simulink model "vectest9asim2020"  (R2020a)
settings: Solver=FixedStepAuto  StartTime=0.0  StopTime=t(end)  FixedStep=dt  RelTol=1e-3  EnableMultiTasking=on
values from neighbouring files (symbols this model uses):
  arm = vectest9kinematics(arm,ind)    [vectest10demo2021.m]    (also in vectest11ademo2021.m; vectest11demo2021.m; vectest9ademo2.m = vectest9kinematics3(arm,ind); vectest9asim2020demo.m = vectest9kinematics3(arm,ind))
  dt = 0.001    [vectest9ademo2.m]    (also in vectest9asim2020demo.m; mobile10demo.m = 0.1; mobile2demo2021.m = 1)
undefined symbols (not defined in the file or in its folder): deg, kg, m, N, s, X, Y, Z
libraries: sm_lib x18, nesl_utility x12

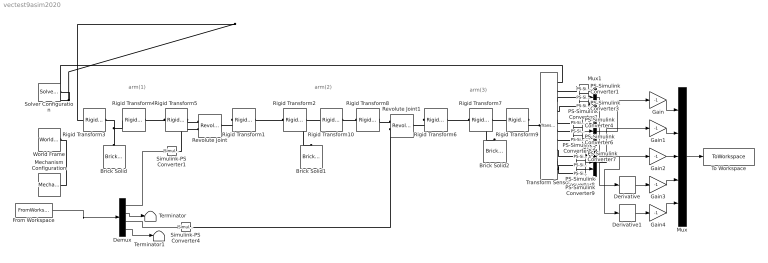
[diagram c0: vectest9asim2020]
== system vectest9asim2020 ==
  note: arm(1)
  note: arm(2)
  note: arm(3)
  Brick Solid : sm_lib/Body Elements/Brick Solid  GraphicAmbientColor=[0.15 0.15 0.15 1.0]  BasedOnType=Density  BrickDimensions=arm(1).l+[0.1;0.1;0]  BrickDimensionUnits=m  CenterOfMass=[0 0 0]  CenterOfMassUnits=m  GraphicDiffuseColor=[0.5 0.5 0.5]  Density=0  DensityUnits=kg/m^3  DoExposeReferenceFrame=on  GraphicEmissiveColor=[0.0 0.0 0.0 1.0]  ExportEntireGeometry=off  SerializedFrames=<Frames/>  MarkerShape=Sphere  MarkerSize=10  GraphicType=FromGeometry  InertiaType=CalculateFromGeometry  Mass=1  MassUnits=kg  MomentsOfInertia=[1 1 1]  MomentsOfInertiaUnits=kg*m^2  GraphicOpacity=1.0  ProductsOfInertia=[0 0 0]  ProductsOfInertiaUnits=kg*m^2  GraphicShininess=75  GraphicSpecularColor=[0.5 0.5 0.5 1.0]  GraphicVisPropType=SimpleVisualProperties
  Brick Solid1 : sm_lib/Body Elements/Brick Solid  GraphicAmbientColor=[0.15 0.15 0.15 1.0]  BasedOnType=Density  BrickDimensions=arm(2).l+[0.1;0.1;0]  BrickDimensionUnits=m  CenterOfMass=[0 0 0]  CenterOfMassUnits=m  GraphicDiffuseColor=[0.5 0.5 0.5]  Density=0  DensityUnits=kg/m^3  DoExposeReferenceFrame=on  GraphicEmissiveColor=[0.0 0.0 0.0 1.0]  ExportEntireGeometry=off  SerializedFrames=<Frames/>  MarkerShape=Sphere  MarkerSize=10  GraphicType=FromGeometry  InertiaType=CalculateFromGeometry  Mass=1  MassUnits=kg  MomentsOfInertia=[1 1 1]  MomentsOfInertiaUnits=kg*m^2  GraphicOpacity=1.0  ProductsOfInertia=[0 0 0]  ProductsOfInertiaUnits=kg*m^2  GraphicShininess=75  GraphicSpecularColor=[0.5 0.5 0.5 1.0]  GraphicVisPropType=SimpleVisualProperties
  Brick Solid2 : sm_lib/Body Elements/Brick Solid  GraphicAmbientColor=[0.15 0.15 0.15 1.0]  BasedOnType=Density  BrickDimensions=arm(3).l+[0.1;0.1;0]  BrickDimensionUnits=m  CenterOfMass=[0 0 0]  CenterOfMassUnits=m  GraphicDiffuseColor=[0.5 0.5 0.5]  Density=0  DensityUnits=kg/m^3  DoExposeReferenceFrame=on  GraphicEmissiveColor=[0.0 0.0 0.0 1.0]  ExportEntireGeometry=off  SerializedFrames=<Frames/>  MarkerShape=Sphere  MarkerSize=10  GraphicType=FromGeometry  InertiaType=PointMass  Mass=0  MassUnits=kg  MomentsOfInertia=[1 1 1]  MomentsOfInertiaUnits=kg*m^2  GraphicOpacity=1.0  ProductsOfInertia=[0 0 0]  ProductsOfInertiaUnits=kg*m^2  GraphicShininess=75  GraphicSpecularColor=[0.5 0.5 0.5 1.0]  GraphicVisPropType=SimpleVisualProperties
  Demux : Demux  Outputs=[1,2,1,2]
  Derivative : Derivative
  Derivative1 : Derivative
  From Workspace : FromWorkspace  VariableName=simin  SampleTime=dt
  Gain{,1..4} (5 alike) : Gain  Gain=-1
  Mechanism Configuration : sm_lib/Utilities/Mechanism Configuration  UniformGravity=Constant  GravityVector=[0 0 0]  GravityUnits=m/s^2  LinearizationDelta=0.001
  Mux : Mux  Inputs=[3,3,3,3,3]
  Mux1 : Mux  Inputs=[1,1,1]
  Mux2 : Mux  Inputs=[1,1,1]
  Mux3 : Mux  Inputs=[1,1,1]
  PS-Simulink Converter{1..9} (9 alike) : nesl_utility/PS-Simulink Converter  PhysicalDomain=network_engine_domain  SubClassName=ps_output  LeftPortType=input  RightPortType=output  PseudoPeriodic=off  Frequencies=[]  Unit=inherit  AffineConversion=off
  Revolute Joint : sm_lib/Joints/Revolute Joint  JointMode=Normal  SenseConstraintForce=off  SenseConstraintForceX=off  SenseConstraintForceY=off  SenseConstraintForceZ=off  SenseConstraintTorque=off  SenseConstraintTorqueX=off  SenseConstraintTorqueY=off  SenseConstraintTorqueZ=off  SenseTotalForce=off  SenseTotalForceX=off  SenseTotalForceY=off  SenseTotalForceZ=off  SenseTotalTorque=off  SenseTotalTorqueX=off  SenseTotalTorqueY=off  SenseTotalTorqueZ=off  CompositeWrenchDir=FollowerOnBase  CompositeWrenchFrame=BaseFrame  EquilibriumPosition=0  EquilibriumPositionUnits=rad  SpringStiffness=0  SpringStiffnessUnits=N*m/deg  DampingCoefficient=0  DampingCoefficientUnits=N*m/(deg/s)  TorqueActuationMode=ComputedTorque  MotionActuationMode=InputMotion  SensePosition=off  SenseVelocity=off  SenseAcceleration=off  SenseTorqueForce=off  SenseLowerLimitTorqueForce=off  SenseUpperLimitTorqueForce=off  LowerLimitSpecify=off  LowerLimitBound=-90  LowerLimitBoundUnits=deg  LowerLimitStiffness=1e4  LowerLimitStiffnessUnits=N*m/deg  LowerLimitDamping=10  LowerLimitDampingUnits=N*m/(deg/s)  LowerLimitTransitionRegionWidth=0.1  LowerLimitTransitionRegionWidthUnits=deg  UpperLimitSpecify=off  UpperLimitBound=90  UpperLimitBoundUnits=deg  UpperLimitStiffness=1e4  UpperLimitStiffnessUnits=N*m/deg  UpperLimitDamping=10  UpperLimitDampingUnits=N*m/(deg/s)  UpperLimitTransitionRegionWidth=0.1  UpperLimitTransitionRegionWidthUnits=deg  PositionTargetSpecify=off  PositionTargetPriority=High  PositionTargetValue=0  PositionTargetValueUnits=deg  VelocityTargetSpecify=off  VelocityTargetPriority=High  VelocityTargetValue=0  VelocityTargetValueUnits=deg/s
  Revolute Joint1 : sm_lib/Joints/Revolute Joint  JointMode=Normal  SenseConstraintForce=off  SenseConstraintForceX=off  SenseConstraintForceY=off  SenseConstraintForceZ=off  SenseConstraintTorque=off  SenseConstraintTorqueX=off  SenseConstraintTorqueY=off  SenseConstraintTorqueZ=off  SenseTotalForce=off  SenseTotalForceX=off  SenseTotalForceY=off  SenseTotalForceZ=off  SenseTotalTorque=off  SenseTotalTorqueX=off  SenseTotalTorqueY=off  SenseTotalTorqueZ=off  CompositeWrenchDir=FollowerOnBase  CompositeWrenchFrame=BaseFrame  EquilibriumPosition=0  EquilibriumPositionUnits=rad  SpringStiffness=0  SpringStiffnessUnits=N*m/deg  DampingCoefficient=0  DampingCoefficientUnits=N*m/(deg/s)  TorqueActuationMode=ComputedTorque  MotionActuationMode=InputMotion  SensePosition=off  SenseVelocity=off  SenseAcceleration=off  SenseTorqueForce=off  SenseLowerLimitTorqueForce=off  SenseUpperLimitTorqueForce=off  LowerLimitSpecify=off  LowerLimitBound=-90  LowerLimitBoundUnits=deg  LowerLimitStiffness=1e4  LowerLimitStiffnessUnits=N*m/deg  LowerLimitDamping=10  LowerLimitDampingUnits=N*m/(deg/s)  LowerLimitTransitionRegionWidth=0.1  LowerLimitTransitionRegionWidthUnits=deg  UpperLimitSpecify=off  UpperLimitBound=90  UpperLimitBoundUnits=deg  UpperLimitStiffness=1e4  UpperLimitStiffnessUnits=N*m/deg  UpperLimitDamping=10  UpperLimitDampingUnits=N*m/(deg/s)  UpperLimitTransitionRegionWidth=0.1  UpperLimitTransitionRegionWidthUnits=deg  PositionTargetSpecify=off  PositionTargetPriority=High  PositionTargetValue=0  PositionTargetValueUnits=deg  VelocityTargetSpecify=off  VelocityTargetPriority=High  VelocityTargetValue=0  VelocityTargetValueUnits=deg/s
  Rigid Transform1 : sm_lib/Frames and Transforms/Rigid Transform  TranslationMethod=None  TranslationStandardOffset=0  TranslationLengthUnit=m  TranslationStandardAxis=+Z  TranslationCartesianOffset=[0 0 0]  TranslationROffset=0  TranslationROffsetUnits=m  TranslationZOffset=0  TranslationZOffsetUnits=m  TranslationThetaOffset=0  TranslationThetaOffsetUnits=deg  RotationMethod=StandardAxis  RotationAngleUnits=deg  RotationStandardAxis=+Y  RotationAngle=-90  RotationArbitraryAxis=[0 0 1]  FollAlignAxisA=+X  BaseAlignAxisA=+Y  FollAlignAxisB=+Y  BaseAlignAxisB=+Z  RotationSequenceAxes=FollowerAxes  RotationSequence=XYX  RotationSequenceAngles=[0 0 0]  RotationSequenceAnglesUnits=deg  RotationMatrix=[1 0 0; 0 1 0; 0 0 1]
  Rigid Transform10 : sm_lib/Frames and Transforms/Rigid Transform  TranslationMethod=Cartesian  TranslationStandardOffset=1  TranslationLengthUnit=m  TranslationStandardAxis=+Z  TranslationCartesianOffset=arm(2).l/2  TranslationROffset=0  TranslationROffsetUnits=m  TranslationZOffset=0  TranslationZOffsetUnits=m  TranslationThetaOffset=0  TranslationThetaOffsetUnits=deg  RotationMethod=None  RotationAngleUnits=deg  RotationStandardAxis=+Y  RotationAngle=-90  RotationArbitraryAxis=[0 0 1]  FollAlignAxisA=+X  BaseAlignAxisA=+Y  FollAlignAxisB=+Y  BaseAlignAxisB=+Z  RotationSequenceAxes=FollowerAxes  RotationSequence=XYX  RotationSequenceAngles=[0 0 0]  RotationSequenceAnglesUnits=deg  RotationMatrix=[1 0 0; 0 1 0; 0 0 1]
  Rigid Transform2 : sm_lib/Frames and Transforms/Rigid Transform  TranslationMethod=Cartesian  TranslationStandardOffset=1  TranslationLengthUnit=m  TranslationStandardAxis=+Z  TranslationCartesianOffset=arm(2).l/2  TranslationROffset=0  TranslationROffsetUnits=m  TranslationZOffset=0  TranslationZOffsetUnits=m  TranslationThetaOffset=0  TranslationThetaOffsetUnits=deg  RotationMethod=None  RotationAngleUnits=deg  RotationStandardAxis=+Y  RotationAngle=-90  RotationArbitraryAxis=[0 0 1]  FollAlignAxisA=+X  BaseAlignAxisA=+Y  FollAlignAxisB=+Y  BaseAlignAxisB=+Z  RotationSequenceAxes=FollowerAxes  RotationSequence=XYX  RotationSequenceAngles=[0 0 0]  RotationSequenceAnglesUnits=deg  RotationMatrix=[1 0 0; 0 1 0; 0 0 1]
  Rigid Transform3 : sm_lib/Frames and Transforms/Rigid Transform  TranslationMethod=Cartesian  TranslationStandardOffset=0  TranslationLengthUnit=m  TranslationStandardAxis=+Z  TranslationCartesianOffset=arm(1).l/2  TranslationROffset=0  TranslationROffsetUnits=m  TranslationZOffset=0  TranslationZOffsetUnits=m  TranslationThetaOffset=0  TranslationThetaOffsetUnits=deg  RotationMethod=None  RotationAngleUnits=deg  RotationStandardAxis=+Y  RotationAngle=-90  RotationArbitraryAxis=[0 0 1]  FollAlignAxisA=+X  BaseAlignAxisA=+Y  FollAlignAxisB=+Y  BaseAlignAxisB=+Z  RotationSequenceAxes=FollowerAxes  RotationSequence=XYX  RotationSequenceAngles=[0 0 0]  RotationSequenceAnglesUnits=deg  RotationMatrix=[1 0 0; 0 1 0; 0 0 1]
  Rigid Transform4 : sm_lib/Frames and Transforms/Rigid Transform  TranslationMethod=Cartesian  TranslationStandardOffset=0  TranslationLengthUnit=m  TranslationStandardAxis=+Z  TranslationCartesianOffset=arm(1).l/2  TranslationROffset=0  TranslationROffsetUnits=m  TranslationZOffset=0  TranslationZOffsetUnits=m  TranslationThetaOffset=0  TranslationThetaOffsetUnits=deg  RotationMethod=None  RotationAngleUnits=deg  RotationStandardAxis=+Y  RotationAngle=-90  RotationArbitraryAxis=[0 0 1]  FollAlignAxisA=+X  BaseAlignAxisA=+Y  FollAlignAxisB=+Y  BaseAlignAxisB=+Z  RotationSequenceAxes=FollowerAxes  RotationSequence=XYX  RotationSequenceAngles=[0 0 0]  RotationSequenceAnglesUnits=deg  RotationMatrix=[1 0 0; 0 1 0; 0 0 1]
  Rigid Transform5 : sm_lib/Frames and Transforms/Rigid Transform  TranslationMethod=None  TranslationStandardOffset=0  TranslationLengthUnit=m  TranslationStandardAxis=+Z  TranslationCartesianOffset=[0 0 0.5]  TranslationROffset=0  TranslationROffsetUnits=m  TranslationZOffset=0  TranslationZOffsetUnits=m  TranslationThetaOffset=0  TranslationThetaOffsetUnits=deg  RotationMethod=StandardAxis  RotationAngleUnits=deg  RotationStandardAxis=+Y  RotationAngle=90  RotationArbitraryAxis=[0 0 1]  FollAlignAxisA=+X  BaseAlignAxisA=+Y  FollAlignAxisB=+Y  BaseAlignAxisB=+Z  RotationSequenceAxes=FollowerAxes  RotationSequence=XYX  RotationSequenceAngles=[0 0 0]  RotationSequenceAnglesUnits=deg  RotationMatrix=[1 0 0; 0 1 0; 0 0 1]
  Rigid Transform6 : sm_lib/Frames and Transforms/Rigid Transform  TranslationMethod=None  TranslationStandardOffset=0  TranslationLengthUnit=m  TranslationStandardAxis=+Z  TranslationCartesianOffset=[0 0 0]  TranslationROffset=0  TranslationROffsetUnits=m  TranslationZOffset=0  TranslationZOffsetUnits=m  TranslationThetaOffset=0  TranslationThetaOffsetUnits=deg  RotationMethod=StandardAxis  RotationAngleUnits=deg  RotationStandardAxis=-X  RotationAngle=-90  RotationArbitraryAxis=[0 0 1]  FollAlignAxisA=+X  BaseAlignAxisA=+Y  FollAlignAxisB=+Y  BaseAlignAxisB=+Z  RotationSequenceAxes=FollowerAxes  RotationSequence=XYX  RotationSequenceAngles=[0 0 0]  RotationSequenceAnglesUnits=deg  RotationMatrix=[1 0 0; 0 1 0; 0 0 1]
  Rigid Transform7 : sm_lib/Frames and Transforms/Rigid Transform  TranslationMethod=Cartesian  TranslationStandardOffset=1  TranslationLengthUnit=m  TranslationStandardAxis=+Z  TranslationCartesianOffset=arm(3).l/2  TranslationROffset=0  TranslationROffsetUnits=m  TranslationZOffset=0  TranslationZOffsetUnits=m  TranslationThetaOffset=0  TranslationThetaOffsetUnits=deg  RotationMethod=None  RotationAngleUnits=deg  RotationStandardAxis=+Y  RotationAngle=-90  RotationArbitraryAxis=[0 0 1]  FollAlignAxisA=+X  BaseAlignAxisA=+Y  FollAlignAxisB=+Y  BaseAlignAxisB=+Z  RotationSequenceAxes=FollowerAxes  RotationSequence=XYX  RotationSequenceAngles=[0 0 0]  RotationSequenceAnglesUnits=deg  RotationMatrix=[1 0 0; 0 1 0; 0 0 1]
  Rigid Transform8 : sm_lib/Frames and Transforms/Rigid Transform  TranslationMethod=None  TranslationStandardOffset=0  TranslationLengthUnit=m  TranslationStandardAxis=+Z  TranslationCartesianOffset=[0 0 0.5]  TranslationROffset=0  TranslationROffsetUnits=m  TranslationZOffset=0  TranslationZOffsetUnits=m  TranslationThetaOffset=0  TranslationThetaOffsetUnits=deg  RotationMethod=StandardAxis  RotationAngleUnits=deg  RotationStandardAxis=-X  RotationAngle=90  RotationArbitraryAxis=[0 0 1]  FollAlignAxisA=+X  BaseAlignAxisA=+Y  FollAlignAxisB=+Y  BaseAlignAxisB=+Z  RotationSequenceAxes=FollowerAxes  RotationSequence=XYX  RotationSequenceAngles=[0 0 0]  RotationSequenceAnglesUnits=deg  RotationMatrix=[1 0 0; 0 1 0; 0 0 1]
  Rigid Transform9 : sm_lib/Frames and Transforms/Rigid Transform  TranslationMethod=Cartesian  TranslationStandardOffset=1  TranslationLengthUnit=m  TranslationStandardAxis=+Z  TranslationCartesianOffset=arm(3).l/2  TranslationROffset=0  TranslationROffsetUnits=m  TranslationZOffset=0  TranslationZOffsetUnits=m  TranslationThetaOffset=0  TranslationThetaOffsetUnits=deg  RotationMethod=None  RotationAngleUnits=deg  RotationStandardAxis=+Y  RotationAngle=-90  RotationArbitraryAxis=[0 0 1]  FollAlignAxisA=+X  BaseAlignAxisA=+Y  FollAlignAxisB=+Y  BaseAlignAxisB=+Z  RotationSequenceAxes=FollowerAxes  RotationSequence=XYX  RotationSequenceAngles=[0 0 0]  RotationSequenceAnglesUnits=deg  RotationMatrix=[1 0 0; 0 1 0; 0 0 1]
  Simulink-PS Converter1 : nesl_utility/Simulink-PS Converter  PhysicalDomain=network_engine_domain  SubClassName=ps_input  LeftPortType=input  RightPortType=output  PseudoPeriodic=off  Frequencies=[]  NoiseDistribution=none  NoiseParameters=[]  Unit=1  AffineConversion=off  FilteringAndDerivatives=filter  SimscapeFilterOrder=2  InputFilterTimeConstant=0.001  UdotUserProvided=0
  Simulink-PS Converter4 : nesl_utility/Simulink-PS Converter  PhysicalDomain=network_engine_domain  SubClassName=ps_input  LeftPortType=input  RightPortType=output  PseudoPeriodic=off  Frequencies=[]  NoiseDistribution=none  NoiseParameters=[]  Unit=1  AffineConversion=off  FilteringAndDerivatives=filter  SimscapeFilterOrder=2  InputFilterTimeConstant=0.001  UdotUserProvided=0
  Solver Configuration : nesl_utility/Solver Configuration  PhysicalDomain=network_engine_domain  SubClassName=solver  LeftPortType=input  RightPortType=generic  Tones=[]  Harmonics=[]  SimulateNoise=off  Profile=off  UseLocalSampling=off  EnableSwitchedLinearOptims=on  FrequencyDomain=off  UseCCode=off  RelTol=0.001  AbsTol=1e-06  MinStep=1e-09  ToWorkspace=off  RevertToSquareIcSolve=off  NumHomotopyIterations=100  PhasorMode=off  PhasorModeNumHarmonics=1  DoDC=off  ResidualTolerance=1e-09  UseLocalSolver=off  LocalSolverChoice=NE_BACKWARD_EULER_ADVANCER  LocalSolverSampleTime=0.001  DoFixedCost=off  MaxNonlinIter=3  MaxModeIter=2  LinearAlgebra=Sparse  EquationFormulation=NE_TIME_EF  DelaysMemoryBudget=1024  AutomaticFiltering=on  FilteringTimeConstant=0.001  PartitionStorageMethod=AS_NEEDED  PartitionMemoryBudget=1024  PartitionMethod=FAST
  Terminator : Terminator
  Terminator1 : Terminator
  To Workspace : ToWorkspace  VariableName=simout1  SaveFormat=Timeseries  SampleTime=-1
  Transform Sensor : sm_lib/Frames and Transforms/Transform Sensor  MeasurementFrame=World  SenseAngle=off  SenseAxis=off  SenseAngle1=off  SenseAngle2=off  SenseAngle3=off  SenseQ=off  SenseR=off  SenseOmegaX=on  SenseOmegaY=on  SenseOmegaZ=on  SenseOmega1=off  SenseOmega2=off  SenseOmega3=off  SenseQDot=off  SenseRDot=off  SenseAlphaX=off  SenseAlphaY=off  SenseAlphaZ=off  SenseAlpha1=off  SenseAlpha2=off  SenseAlpha3=off  SenseQDDot=off  SenseRDDot=off  SenseX=on  SenseY=on  SenseZ=on  SenseRad=off  SenseAzim=off  SenseDist=off  SenseInc=off  SenseXDot=on  SenseYDot=on  SenseZDot=on  SenseRadDot=off  SenseAzimDot=off  SenseDistDot=off  SenseIncDot=off  SenseXDDot=off  SenseYDDot=off  SenseZDDot=off  SenseRadDDot=off  SenseAzimDDot=off  SenseDistDDot=off  SenseIncDDot=off
  World Frame : sm_lib/Frames and Transforms/World Frame
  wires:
  From Workspace/1 -> Demux/1
  Demux/1 -> Simulink-PS Converter1/1
  Mux/1 -> To Workspace/1
  Demux/3 -> Simulink-PS Converter4/1
  Demux/2 -> Terminator/1
  Demux/4 -> Terminator1/1
  PS-Simulink Converter1/1 -> Mux1/1
  PS-Simulink Converter2/1 -> Mux1/2
  PS-Simulink Converter3/1 -> Mux1/3
  PS-Simulink Converter4/1 -> Mux2/1
  PS-Simulink Converter5/1 -> Mux2/2
  PS-Simulink Converter6/1 -> Mux2/3
  PS-Simulink Converter9/1 -> Mux3/3
  PS-Simulink Converter8/1 -> Mux3/2
  PS-Simulink Converter7/1 -> Mux3/1
  Gain/1 -> Mux/1
  Gain1/1 -> Mux/2
  Gain2/1 -> Mux/3
  Gain3/1 -> Mux/4
  Gain4/1 -> Mux/5
  Mux2/1 -> Gain/1
  Mux3/1 -> Derivative/1, Gain1/1
  Derivative1/1 -> Gain4/1
  Derivative/1 -> Gain3/1
  Mux1/1 -> Derivative1/1, Gain2/1
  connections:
  Simulink-PS Converter1/RConn1 -- Revolute Joint/LConn2
  Rigid Transform1/LConn1 -- Revolute Joint/RConn1
  Rigid Transform1/RConn1 -- Rigid Transform2/LConn1
  Rigid Transform5/RConn1 -- Revolute Joint/LConn1
  Rigid Transform2/RConn1 -- Rigid Transform10/LConn1 -- Brick Solid1/RConn1
  Rigid Transform7/RConn1 -- Rigid Transform9/LConn1 -- Brick Solid2/RConn1
  Rigid Transform8/RConn1 -- Revolute Joint1/LConn1
  Rigid Transform6/LConn1 -- Revolute Joint1/RConn1
  Rigid Transform6/RConn1 -- Rigid Transform7/LConn1
  Revolute Joint1/LConn2 -- Simulink-PS Converter4/RConn1
  Rigid Transform9/RConn1 -- Transform Sensor/LConn1
  PS-Simulink Converter1/LConn1 -- Transform Sensor/RConn2
  Transform Sensor/RConn3 -- PS-Simulink Converter2/LConn1
  Transform Sensor/RConn4 -- PS-Simulink Converter3/LConn1
  Rigid Transform5/LConn1 -- Rigid Transform4/RConn1
  Brick Solid/RConn1 -- Rigid Transform4/LConn1 -- Rigid Transform3/RConn1
  World Frame/RConn1 -- Mechanism Configuration/RConn1 -- Transform Sensor/RConn1 -- Solver Configuration/RConn1 -- Rigid Transform3/LConn1
  Rigid Transform8/LConn1 -- Rigid Transform10/RConn1
  Transform Sensor/RConn5 -- PS-Simulink Converter4/LConn1
  Transform Sensor/RConn7 -- PS-Simulink Converter6/LConn1
  Transform Sensor/RConn6 -- PS-Simulink Converter5/LConn1
  Transform Sensor/RConn8 -- PS-Simulink Converter7/LConn1
  Transform Sensor/RConn10 -- PS-Simulink Converter9/LConn1
  Transform Sensor/RConn9 -- PS-Simulink Converter8/LConn1
